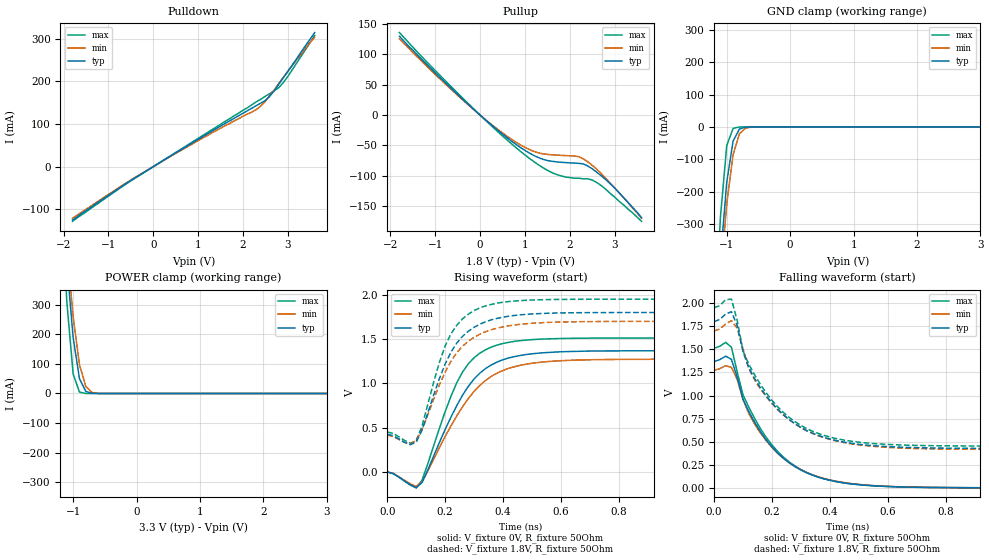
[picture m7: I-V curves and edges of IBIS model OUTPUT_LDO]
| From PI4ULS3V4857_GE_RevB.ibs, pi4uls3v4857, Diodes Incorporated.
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| Model  OUTPUT
[Model]  OUTPUT_LDO
Model_type  Output
Vmeas=0.9
|Variable   typ   min   max
C_comp   8.10p   8.03p   8.15p
|Variable   typ   min   max
[Voltage Range]   1.8   1.7   1.95
[Temperature Range]   40   85   -40
[Pullup Reference]   1.8   1.7   1.95
[Pulldown Reference]   0   0   0
[Power Clamp Reference]   3.3   2.9   3.6
[GND Clamp Reference]   0   0   0
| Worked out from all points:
|   slope of the pulldown table from 0 to 0.27 V, typ, clamps not added: 15.5 ohm
|   slope of the pullup table from 0 to 0.27 V, typ, clamps not added: 15.5 ohm
|   GND clamp passes 1 mA (typ) near -0.71 V on its own axis
|   POWER clamp passes 1 mA (typ) near -0.71 V on its own axis
|   falling waveform, V_fixture 0V, R_fixture 50Ohm: 20-80 % time 170ps typ, 174ps min, 168ps max; typ from 1.37 V to 0 V
|   falling waveform, V_fixture 1.8V, R_fixture 50Ohm: 20-80 % time 180ps typ, 184ps min, 175ps max; typ from 1.8 V to 0.426 V
|   rising waveform, V_fixture 0V, R_fixture 50Ohm: 20-80 % time 141ps typ, 157ps min, 117ps max; typ from 0 V to 1.37 V
|   rising waveform, V_fixture 1.8V, R_fixture 50Ohm: 20-80 % time 115ps typ, 125ps min, 99.9ps max; typ from 0.426 V to 1.8 V
[GND Clamp]
-3.3V     -9.7A      -8.62A     -12.6A
-1.1V     -409mA     -469mA     -279mA
-1V       -170mA     -237mA     -57.3mA
-800mV    -6.62mA    -20.8mA    -103uA
3.6V      258pA      3.3mA      21.6pA
3.9V      13.9uA     259mA      25.2pA
4.1V      6.95mA     782mA      60.1pA
4.4V      440mA      1.77A      78.5uA
4.5V      761mA      2.12A      4.66mA
4.6V      1.12A      2.48A      66.1mA
4.7V      1.5A       2.84A      311mA
6.6V      9.7A       10.1A      11.2A
[POWER Clamp]
-3.3V     9.7A       8.51A      13.1A
-1.2V     761mA      782mA      723mA
-1.1V     440mA      496mA      311mA
-1V       189mA      259mA      66.1mA
-900mV    49.7mA     97mA       4.66mA
-600mV    13.9uA     243uA      4.57nA
3.6V      -380pA     -3.34mA    -21.6pA
4.1V      -6.62mA    -754mA     -77.4pA
4.4V      -409mA     -1.75A     -103uA
4.5V      -725mA     -2.11A     -4.58mA
4.8V      -1.86A     -3.21A     -669mA
6.6V      -9.7A      -10.2A     -10.8A
[Pulldown]
| Voltage   I(typ)   I(min)  I(max)
-1.8V     -125mA     -121mA     -128mA
-400mV    -25.9mA    -25mA      -26.6mA
1.1V      70.2mA     66.9mA     72.8mA
2.3V      143mA      134mA      152mA
2.4V      149mA      142mA      158mA
2.5V      155mA      153mA      165mA
2.6V      165mA      167mA      171mA
2.8V      193mA      195mA      185mA
2.9V      208mA      209mA      197mA
3V        223mA      223mA      211mA
3.4V      284mA      278mA      275mA
3.6V      314mA      303mA      307mA
[Pullup]   |Note: Vtable = Vcc - Voutput
| Voltage   I(typ)   I(min)  I(max)
-1.8V     130mA      126mA      136mA
-100mV    6.66mA     6.34mA     7.13mA
500mV     -31.5mA    -29.5mA    -34.4mA
1V        -58.1mA    -53.2mA    -65.6mA
1.3V      -70mA      -62.2mA    -81.9mA
1.6V      -76.1mA    -65.4mA    -94.7mA
1.9V      -78.2mA    -66.7mA    -102mA
2.3V      -80.4mA    -72.1mA    -105mA
2.5V      -88.5mA    -82.7mA    -107mA
2.7V      -100mA     -96.2mA    -116mA
3V        -120mA     -120mA     -135mA
3.6V      -169mA     -170mA     -175mA
[Falling Waveform]
V_fixture = 0V
V_fixture_min = 0V
V_fixture_max = 0V
R_fixture = 50Ohm
C_fixture = 0F
|   Time   V(typ)   V(min)   V(max)
0s        1.368V     1.273V     1.512V
40ps      1.426V     1.323V     1.576V
60ps      1.392V     1.306V     1.523V
100ps     960.5mV    955.6mV    1.006V
140ps     712mV      692.4mV    752mV
200ps     443.2mV    437mV      464.3mV
280ps     229.3mV    229.9mV    235.9mV
400ps     81.99mV    85.77mV    82.5mV
700ps     6.53mV     7.315mV    6.237mV
1.98ns    27.19uV    38.51uV    17.58uV
[Falling Waveform]
V_fixture = 1.8V
V_fixture_min = 1.7V
V_fixture_max = 1.95V
R_fixture = 50Ohm
C_fixture = 0F
|   Time   V(typ)   V(min)   V(max)
0s        1.8V       1.7V       1.95V
60ps      1.907V     1.811V     2.044V
80ps      1.757V     1.727V     1.81V
100ps     1.473V     1.503V     1.485V
120ps     1.299V     1.294V     1.338V
220ps     851.2mV    845.7mV    877.1mV
300ps     653.8mV    652mV      675.4mV
420ps     513.5mV    509.8mV    534.7mV
720ps     434.2mV    424.2mV    458.5mV
1.98ns    426.2mV    415.1mV    451.5mV
[Rising Waveform]
V_fixture = 0V
V_fixture_min = 0V
V_fixture_max = 0V
R_fixture = 50Ohm
C_fixture = 0F
|   Time   V(typ)   V(min)   V(max)
0s        0V         0V         0V
100ps     -179mV     -164.2mV   -179.2mV
120ps     -119.3mV   -111.1mV   -92.95mV
200ps     479.8mV    400.4mV    680.5mV
260ps     866.2mV    735.9mV    1.127V
320ps     1.116V     978.6mV    1.341V
400ps     1.267V     1.146V     1.45V
500ps     1.333V     1.227V     1.493V
660ps     1.361V     1.263V     1.509V
1.98ns    1.368V     1.273V     1.512V
[Rising Waveform]
V_fixture = 1.8V
V_fixture_min = 1.7V
V_fixture_max = 1.95V
R_fixture = 50Ohm
C_fixture = 0F
|   Time   V(typ)   V(min)   V(max)
0s        426.2mV    415mV      451.4mV
80ps      307.9mV    317.7mV    323.9mV
100ps     337.5mV    357.9mV    353.4mV
120ps     470.5mV    476.7mV    518.3mV
180ps     1.053V     980.9mV    1.236V
220ps     1.352V     1.248V     1.558V
280ps     1.588V     1.475V     1.78V
360ps     1.717V     1.606V     1.891V
600ps     1.794V     1.692V     1.947V
1.98ns    1.8V       1.7V       1.95V
[Ramp]
|   typ   min   max
dV/dt_r   1.24/1.04E-10   1.15/1.16E-10   1.35/0.86E-10
dV/dt_f   1.14/1.74E-10   1.06/1.77E-10   1.26/1.73E-10
R_load =   50.0000
